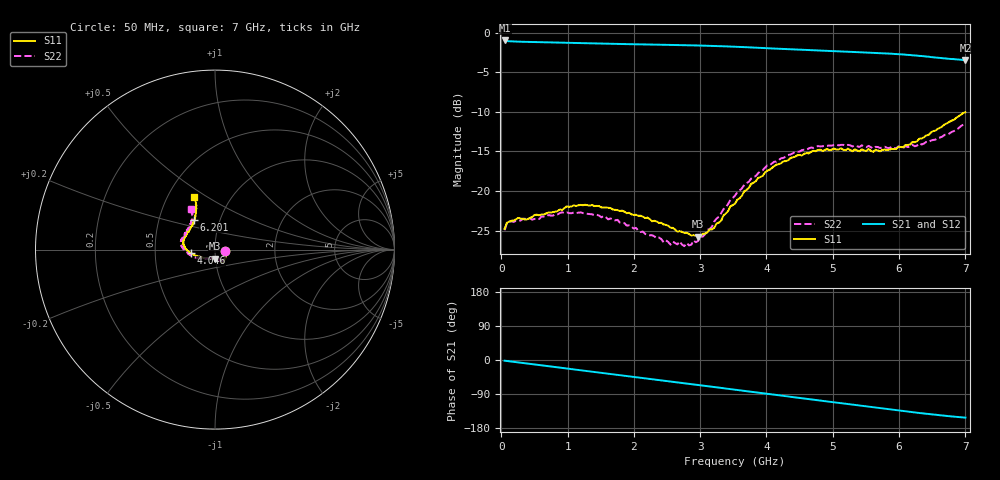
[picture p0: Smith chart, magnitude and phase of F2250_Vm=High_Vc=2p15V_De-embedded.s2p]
! Integrated Device Technology
! Corporate Headquarters
! 6024 Silver Creek Valley Road
! San Jose, CA 95138  USA
! Phone:  1-408-284-8200
! Toll Free:  1-800-223-1366
! Webpage:  http://www.idt.com/
! Timing and RF Division
! 515 Groton Road, Suite 102
! Westford, MA 01886-6024
! Device:  F2250
! Description: Voltage Variable RF Attenuator
! Frequency:  50.0 -  6000.00 MHz
! Package:  3x3 mm Thin QFN Plastic Package: 16 pin
! Ports:  2 RF, 3 DC
!  Pin  1  = GND
!  Pin  2  = NC
!  Pin  3  = RF1  = Port 1
!  Pin  4  = NC
!  Pin  5  = GND
!  Pin  6  = GND
!  Pin  7  = GND
!  Pin  8  = GND
!  Pin  9  = NC
!  Pin 10  = RF2  = Port 2
!  Pin 11  = NC
!  Pin 12  = GND
!  Pin 13  = GND
!  Pin 14  = VCNTRL
!  Pin 15  = VDD
!  Pin 16  = VMODE
! Vcntrl:  2.150 Volts
! Vmode:  +3.300 Volts
! Vdd:  +3.30  Volts
! Current:  1.319 mA
! Data:  The device was measured on a the F2250 evaluation board which has
!  individual transmission lines to the RF pins.  Data was collected
!  using a calibrated network analyzer.  The evaluation board was
!  de-embedded using a TRL calibration technique.
!  The reference plane is the edge of the package pin.
! Misc:  SN 10
!  Action Tracker AT0258
! Date Measured:  2014-11-26
! Date:  2015-10-15  MJV
! Note:
!  Integrated Device Technology supplies this data as a sample of measured
!  data at the package pin for this product.  Your particular data for this
!  product may vary.
!  Data was taken at 25 degrees C.
!  Integrated Device Technology reserves the right to change this data at anytime.
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# GHz S dB R 50
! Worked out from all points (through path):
!   201 points, 50 MHz to 7 GHz, reference 50 ohm
!   highest |S21| = -0.94 dB at 50 MHz (marker M1); lowest = -3.4 dB at 7 GHz (marker M2)
!   group delay of S21, straight-line fit = 61.1 ps
!   lowest |S11| = -25.8 dB at 2.969 GHz (marker M3), VSWR 1.11, Z = 49.5 - j5.1 ohm
!   |S11| at or under -10 dB: start of sweep to end of sweep
!   |S22| runs from -27.0 to -11.5 dB; largest |S21 - S12| = 0.0019
!   S11 on the Smith chart (normalised r, x): 50 MHz: 1.12, -0.02; 4.046 GHz: 0.76, -0.03; 6.201 GHz: 0.75, +0.26; 7 GHz: 0.68, +0.44
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0.05  -24.77 -9.7  -0.94 -1.8  -0.94 -1.8  -24.97 -10.1
0.08475  -24.00 -8.8  -1.01 -2.5  -1.01 -2.5  -24.05 -9.0
0.1195  -23.89 -9.4  -1.04 -3.3  -1.04 -3.2  -23.87 -8.4
0.91875  -22.39 -47.3  -1.23 -21.0  -1.23 -21.1  -22.69 -49.4
1.2315  -21.80 -55.1  -1.30 -27.9  -1.30 -27.9  -22.80 -59.8
1.75275  -22.42 -62.0  -1.39 -39.1  -1.39 -39.1  -23.65 -66.9
2.37825  -24.04 -62.1  -1.48 -52.8  -1.48 -52.8  -25.89 -68.2
2.552  -24.65 -66.6  -1.50 -56.6  -1.50 -56.7  -26.79 -74.7
2.691  -25.07 -74.1  -1.53 -59.7  -1.53 -59.7  -26.38 -82.0
2.7605  -25.31 -76.0  -1.54 -61.3  -1.54 -61.3  -26.98 -86.4
2.969  -25.78 -92.6  -1.58 -66.0  -1.58 -66.0  -26.32 -104.6
3.21225  -24.64 -122.3  -1.64 -71.4  -1.64 -71.5  -23.85 -128.9
3.525  -21.61 -148.7  -1.74 -78.5  -1.74 -78.5  -20.60 -147.5
3.76825  -19.10 -161.8  -1.83 -84.0  -1.83 -84.0  -18.43 -158.6
4.04625  -17.32 -171.7  -1.94 -90.2  -1.94 -90.2  -16.74 -169.1
4.4285  -15.69 177.8  -2.08 -98.6  -2.09 -98.6  -15.05 179.3
4.7065  -14.91 170.7  -2.18 -104.8  -2.19 -104.8  -14.55 173.5
5.054  -14.76 162.5  -2.31 -112.4  -2.31 -112.5  -14.15 166.4
5.85325  -14.77 136.5  -2.61 -130.0  -2.61 -130.1  -14.56 147.5
6.20075  -13.81 124.7  -2.82 -137.7  -2.82 -137.8  -14.15 138.5
6.54825  -12.36 116.5  -3.09 -144.7  -3.09 -144.8  -13.50 127.1
7  -10.04 111.5  -3.42 -152.0  -3.43 -152.2  -11.49 120.8
